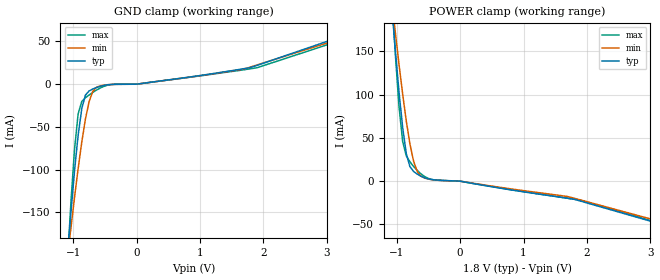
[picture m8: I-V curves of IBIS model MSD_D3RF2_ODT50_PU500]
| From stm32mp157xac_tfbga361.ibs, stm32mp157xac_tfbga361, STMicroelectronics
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[Model] MSD_D3RF2_ODT50_PU500
Model_type   Input
C_comp 2.300pF   2.262pF   2.329pF
Vinh = 1.150V
Vinl = 650.000mV
[Model Spec]
Vinh   1.150V   1.100V   1.200V
Vinl   650.000mV   600.000mV   700.000mV
[Temperature Range]   25.000   125.000   -40.000
[Voltage Range]   1.800V   1.700V   1.900V
[GND Clamp Reference]   0.00V   0.00V   0.00V
[POWER Clamp Reference]   1.800V   1.700V   1.900V
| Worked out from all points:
|   GND clamp passes 1 mA (typ) near -0.48 V on its own axis
|   POWER clamp passes 1 mA (typ) near -0.31 V on its own axis
[GND Clamp]
-1.785V   -919.7mA   -680.2mA   -1.29A
-1.094V   -204.9mA   -206.3mA   -215.1mA
-1.036V   -151.2mA   -169.1mA   -139.8mA
-978.8mV  -102.1mA   -133.1mA   -76.83mA
-921.2mV  -59.78mA   -98.96mA   -34.7mA
-863.6mV  -28.46mA   -67.6mA    -20.2mA
-806.1mV  -12.77mA   -40.74mA   -15.86mA
-748.5mV  -7.878mA   -20.4mA    -12.63mA
-690.9mV  -5.662mA   -8.512mA   -9.668mA
-575.8mV  -2.57mA    -1.96mA    -4.56mA
1.785V    19.34mA    19.88mA    17.92mA
3.57V     64.57mA    61.42mA    59.89mA
[Power Clamp]
-1.77V    921.3mA    689.3mA    1.288A
-1.079V   202.8mA    209.1mA    217.8mA
-1.021V   150.5mA    171.5mA    146.5mA
-963.6mV  103.1mA    135.1mA    86.21mA
-906.1mV  62.12mA    100.6mA    45.93mA
-848.5mV  31.77mA    69.32mA    29.2mA
-790.9mV  16.66mA    42.77mA    22.27mA
-733.3mV  11.16mA    22.89mA    16.96mA
-618.2mV  5.704mA    5.76mA     8.476mA
-445.5mV  1.822mA    1.703mA    1.845mA
1.8V      -21mA      -19.83mA   -20.98mA
3.585V    -58.63mA   -55.29mA   -58.01mA
